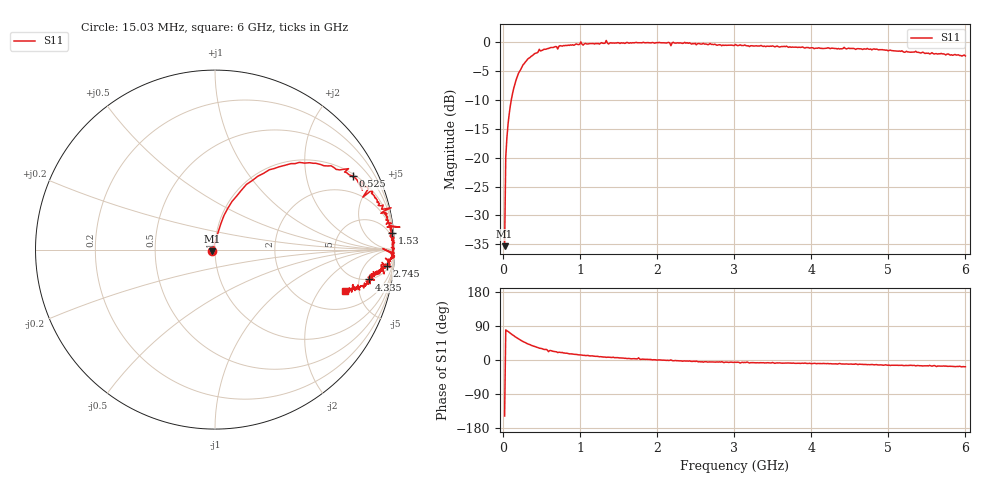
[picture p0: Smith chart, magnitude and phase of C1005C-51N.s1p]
!	Network	Analyzer	HP8753E.07.74:	Oct	30	2002	Serial	No.	JP38451487
!	Hewlett-Packard
!	7	Sep	2009	9:10:34
!	Frequency	S11
#	HZ	S	RI	R	50
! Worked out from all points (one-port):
!   400 points, 15.03 MHz to 6 GHz, reference 50 ohm
!   lowest |S11| = -35.3 dB at 15.03 MHz (marker M1), VSWR 1.03, Z = 48.6 - j0.888 ohm
!   |S11| at or under -10 dB: start of sweep to 101.9 MHz
!   S11 on the Smith chart (normalised r, x): 15.03 MHz: 0.97, -0.02; 525 MHz: 1.10, +3.70; 1.53 GHz: 2, +22; 2.745 GHz: 7, -18; 4.335 GHz: 4.94, -7.04; 6 GHz: 3.25, -3.58
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1.502992e7  -0.0145 -0.00914
3.002985e7  0.0185 0.0999
6.00297e7  0.05 0.19
1.050295e8  0.123 0.301
2.550287e8  0.423 0.479
4.650277e8  0.744 0.451
5.250274e8  0.768 0.409
5.850271e8  0.821 0.331
6.150269e8  0.818 0.379
7.650262e8  0.872 0.314
1.005025e9  0.981 0.233
1.035025e9  0.924 0.202
1.320023e9  0.974 0.133
1.335023e9  1.03 0.125
1.365023e9  0.959 0.126
1.515022e9  0.972 0.0923
1.530022e9  0.987 0.0909
1.755021e9  0.986 0.0997
2.145019e9  0.998 -0.0204
2.175019e9  0.935 0.00513
2.265019e9  0.99 -0.0308
2.745016e9  0.96 -0.0926
3.015015e9  0.952 -0.101
3.765011e9  0.898 -0.127
4.335008e9  0.86 -0.166
4.515007e9  0.871 -0.163
5.265004e9  0.799 -0.205
6e9  0.725 -0.232
